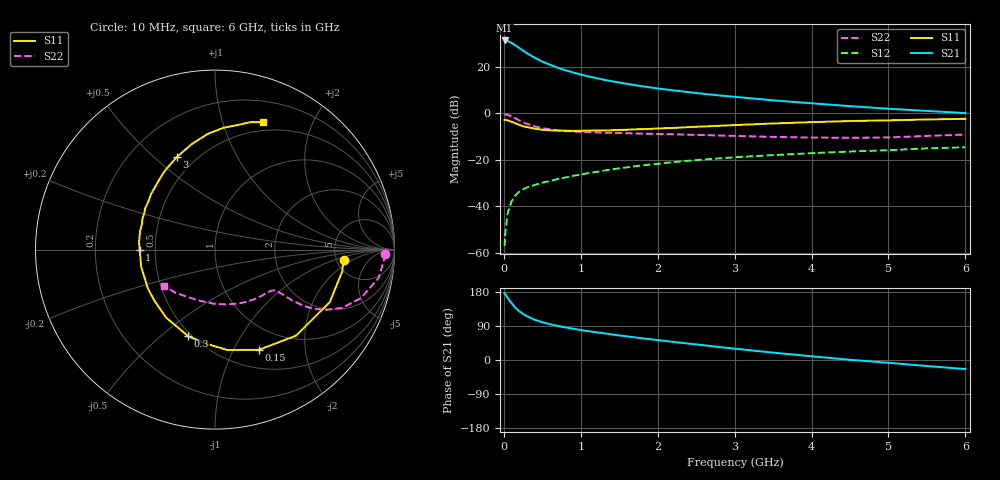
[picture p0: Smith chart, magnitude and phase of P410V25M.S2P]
! SIEMENS Small Signal Semiconductors
! BFP182
! Si NPN RF Bipolar Junction Transistor in SOT143
! VCE = 10 V  IC = 25 mA
! Common Emitter S-Parameters:  March  1996
# GHz  S  MA  R  50
!  f  S11  S21  S12  S22
! GHz  MAG  ANG  MAG  ANG  MAG  ANG  MAG  ANG
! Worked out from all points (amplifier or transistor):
!   36 points, 10 MHz to 6 GHz, reference 50 ohm
!   highest |S21| = 31.3 dB at 10 MHz (marker M1)
!   |S21| within 3 dB of that: start of sweep to 189.5 MHz
!   unconditionally stable (mu >= 1): 857.1 MHz to 5.716 GHz
!   at 250 MHz: K = 0.49, MSG = 29.8 dB, |S12| = -32.7 dB
!   at 1.4 GHz: K = 1.13, MAG = 16.7 dB, |S12| = -24.1 dB
!   at 6 GHz: K = 0.98, MSG = 7.3 dB, |S12| = -14.6 dB
!   S11 on the Smith chart (normalised r, x): 10 MHz: 5.79, -1.35; 150 MHz: 0.71, -1.27; 300 MHz: 0.48, -0.62; 1 GHz: 0.41, -0.00; 3 GHz: 0.40, +0.59; 6 GHz: 0.41, +1.37
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0.01  0.7187 -4.5  36.6 175.7  0.0014 65.6  0.9482 -1.6
0.02  0.7192 -9.7  36.44 173.2  0.0028 78.1  0.9426 -3.7
0.05  0.7031 -24.6  35.66 163.8  0.0072 76.7  0.9258 -9.8
0.1  0.6587 -46.7  32.25 149.9  0.0128 66.0  0.8567 -18.4
0.15  0.6096 -66.3  28.65 138.0  0.0172 62.0  0.7794 -24.6
0.2  0.5638 -82.9  25.22 128.6  0.0209 57.5  0.7042 -28.5
0.25  0.5262 -95.6  22.01 121.3  0.0232 53.7  0.6427 -30.9
0.3  0.5054 -107.2  19.49 115.8  0.0255 52.0  0.5942 -32.2
0.4  0.4665 -125.7  15.6 106.3  0.0288 52.0  0.5233 -33.3
0.5  0.442 -139.6  12.84 99.6  0.0323 50.6  0.4788 -33.5
0.6  0.432 -150.2  11 94.4  0.0352 51.1  0.45 -33.5
0.7  0.422 -159.4  9.467 89.9  0.0385 52.2  0.431 -33.7
0.8  0.4225 -167.2  8.408 85.9  0.0417 52.1  0.4168 -34.0
1  0.42 -179.8  6.764 79.1  0.048 52.9  0.398 -34.8
1.1  0.4251 174.8  6.201 75.9  0.052 52.9  0.3919 -35.7
1.5  0.4389 157.4  4.566 64.8  0.0657 51.9  0.3757 -40.1
2.2  0.4837 133.4  3.102 47.8  0.0893 47.2  0.354 -51.1
3  0.5578 112.5  2.254 29.9  0.1135 40.3  0.3266 -67.3
3.5  0.6035 102.1  1.896 19.5  0.1263 35.4  0.3108 -79.2
4.5  0.6807 86.0  1.421 0.6  0.1507 26.8  0.297 -105.8
5.5  0.736 74.6  1.123 -15.9  0.1762 19.2  0.326 -132.3
6  0.7591 69.2  1.01 -23.9  0.1864 14.5  0.3489 -145.0
